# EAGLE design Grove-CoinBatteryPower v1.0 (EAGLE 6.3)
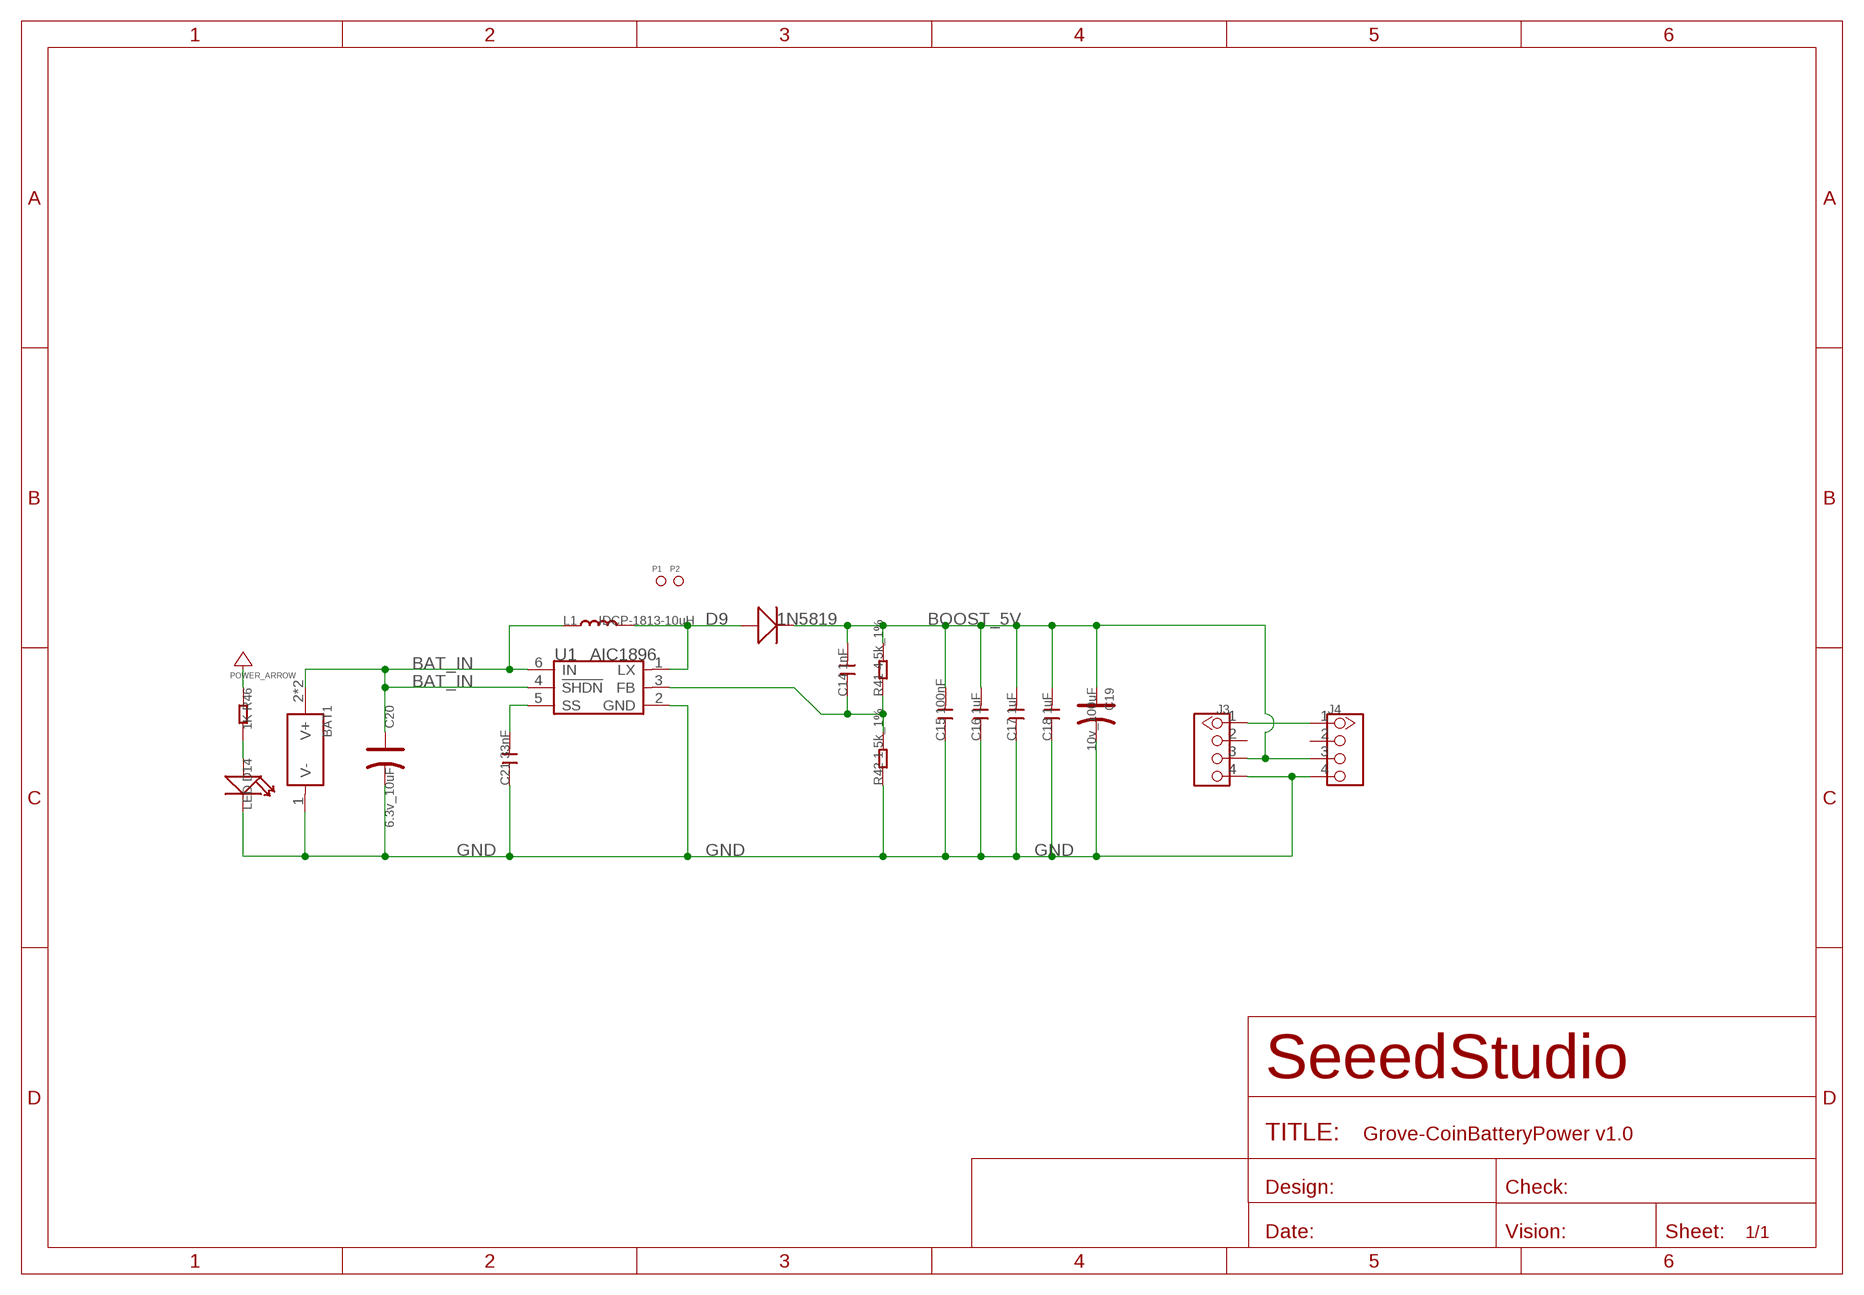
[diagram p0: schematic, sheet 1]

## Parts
BAT1  HOLDER-BAT-CIRCLE  [2032-D20-CIRCLE]
C14  1nF  C-0603  [C0603]
C15  100nF  C-0603  [C0603]
C16  1uF  C-0805  [C0805]
C17  1uF  C-0805  [C0805]
C18  1uF  C-0805  [C0805]
C19  10v_100uF  006-CAP_AVX_C  [AVX_C]
C20  6.3v_10uF  CAP-AVX-A  [AVX-A]
C21  33nF  C-0603  [C0603]
D9  1N5819  D'SMA'  [D2010]
D14  LED  LED'0603'  [LED-0603]
J3  TWIG-4P-2.0'90D'  [4P-2.0-90D]
J4  TWIG-4P-2.0'90D'  [4P-2.0-90D]
L1  IDCP-1813-10uH  013-L1813  [1813@1]
P1  PAD-MARK  [ROUND-MARK-1.0]
P2  PAD-MARK  [ROUND-MARK-1.0]
R41  4.5k_1%  R-0603  [R0603]
R42  1.5k_1%  R-0603  [R0603]
R46  1K  R-0603  [R0603]
U1  AIC1896  [SOT23-6]

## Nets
BAT_IN: BAT1.2(V+) BAT1.3(V+) C20.+ L1.1 U1.4(!SHDN) U1.6(IN)
BOOST_5V: C14.2 C15.2 C16.2 C17.2 C18.2 C19.+ D9.- J3.3 J4.3 R41.2 R46.1 ; supply symbol labelled POWER_ARROW
GND: BAT1.1(V-) C15.1 C16.1 C17.1 C18.1 C19.- C20.- C21.1 D14.- J3.4 J4.4 R42.1 U1.2(GND)
N$3: J3.1 J4.1
N$35: C21.2 U1.5(SS)
N$36: D9.+ L1.2 U1.1(LX)
N$37: C14.1 R41.1 R42.2 U1.3(FB)
N$74: D14.+ R46.2
Unconnected: J3.2 J4.2

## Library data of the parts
BAT1 = Connector:HOLDER-BAT: button cell holder
C14-C18 C21 = Discrete:C*: Ceramic Capacitors
C19 = Discrete:006-CAP*: Electrolytic Capacitors,Tantalum Capacitors and Super Capacitors
C20 = Discrete:CAP*: Electrolytic Capacitors,Tantalum Capacitors and Super Capacitors
D9 = Discrete:D*
D14 = Discrete:LED*
J3 J4 = Connector:TWIG-4P-2.0
L1 = Discrete:013-L*
P1 P2 = Discrete:PAD-MARK; PARTNO: DNP
R41 R42 R46 = Discrete:R*
U1 = ICs_v54:AIC1896

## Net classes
0 default: width 0.152 mm, drill 0.305 mm, clearance 0.152 mm

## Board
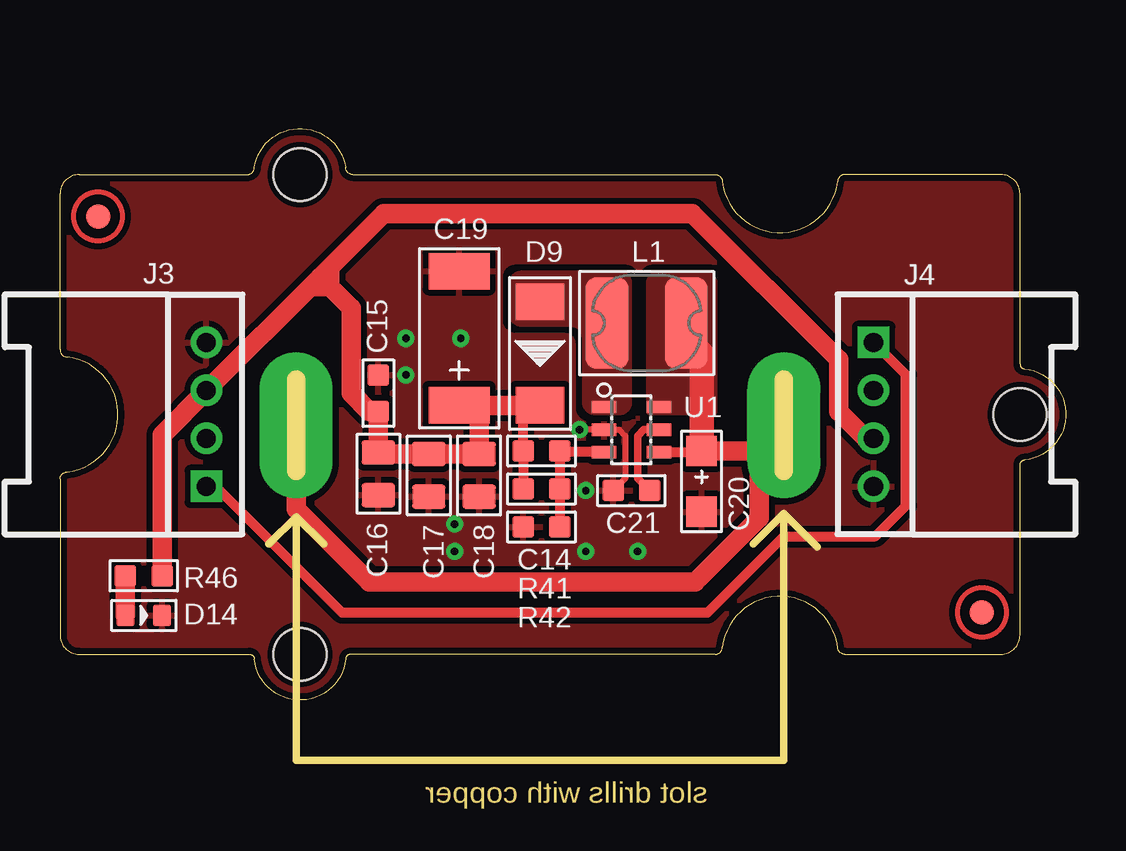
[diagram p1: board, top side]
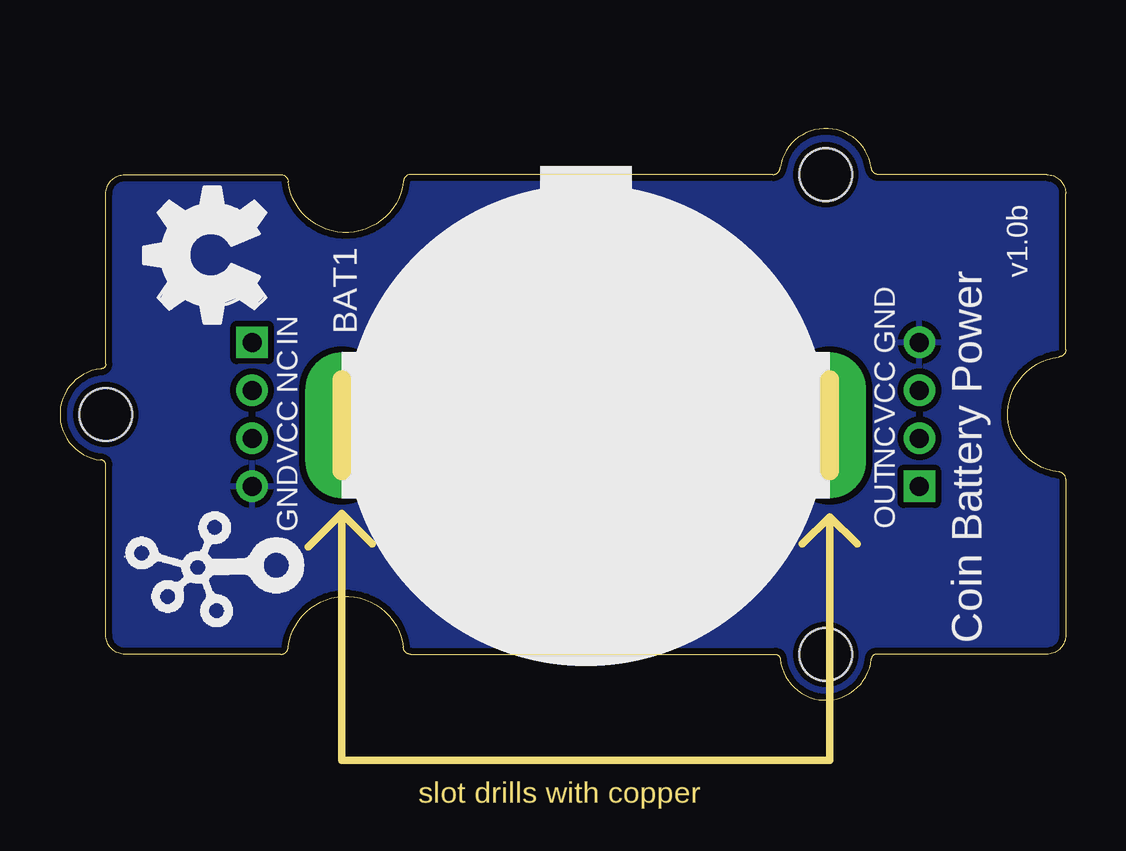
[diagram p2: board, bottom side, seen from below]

Size 41.91 x 23.83 mm. Coordinates in mm from the lower left corner, seen from the top.
Copper layers (1*16): Top 0.035mm / dielectric 1.5mm / Bottom 0.035mm
Design rules "default *": minimum track width 10mil, minimum drill 12mil, track to track 8mil, track to pad 8mil, pad to pad 8mil, via to via 8mil, smd to smd 0mil, copper to edge 10mil, drill to drill 8mil, minimum pad ring 10mil, minimum via ring 8mil, stop-mask expansion 4mil, vias tented up to drill 25mil, thermal gap 10mil

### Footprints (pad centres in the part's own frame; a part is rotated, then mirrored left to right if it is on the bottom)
2032-D20-CIRCLE = smd 15.24 x 15.24: 1 0,0 | drill 0.762 pad 3.048 long: 2 -10.16,0; 3 10.16,0
C0603 = smd 0.889 x 0.889: 1 -0.762,0; 2 0.762,0
C0805 = smd 1.016 x 1.397: 1 -0.889,0; 2 0.889,0
AVX_C = smd 1.524 x 2.54: + -2.794,0; - 2.794,0
AVX-A = smd 1.27 x 1.27: + -1.27,0; - 1.27,0
D2010 = smd 1.524 x 2.032: + -2.159,0; - 2.159,0
LED-0603 = smd 0.762 x 0.889: + -0.762,0; - 0.762,0
4P-2.0-90D = drill 0.8 pad 1.27 square: 1 -3,0 | drill 0.8 pad 1.27: 2 -1,0; 3 1,0; 4 3,0
1813@1 = smd 1.778 x 3.81: 1 -1.651,0; 2 1.651,0
ROUND-MARK-1.0 = smd 1.016 x 1.016: P$1 0,0
R0603 = smd 0.889 x 0.889: 1 -0.762,0; 2 0.762,0
SOT23-6 = smd 0.508 x 1.016: 1 -0.94,-1.143; 2 0,-1.143; 3 0.94,-1.143; 4 0.94,1.143; 5 0,1.143; 6 -0.94,1.143
2U-DIM-W/DRILL = hole 2.2: -10,-10; -10,10; 20,0

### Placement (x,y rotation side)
BAT1  20,11.45 0 bottom
C14  20.06,10.38 180 top
C15  13.27,12.8 270 top
C16  13.27,9.43 90 top
C17  15.36,9.37 90 top
C18  17.46,9.37 90 top
C19  16.63,15.08 90 top
C20  26.73,9.11 270 top
C21  23.81,8.73 0 top
D9  20,14.45 270 top
D14  3.49,3.53 0 top
J3  6.1,11.91 90 top
J4  33.9,11.91 270 top
L1  24.45,15.72 180 top
P1  1.59,20.16 0 top
P2  38.41,3.65 0 top
R41  20.06,8.8 180 top
R42  20.06,7.21 0 top
R46  3.49,5.18 180 top
U1  23.81,11.27 270 top
U$3  [OSHW_FILLX200_NOTEXT]  33.34,15.72 90 bottom
U$4  [TWIGLOGO]  32.7,5.56 90 bottom
U$6  [2U-DIM-W/DRILL]  20,11.91 0 top

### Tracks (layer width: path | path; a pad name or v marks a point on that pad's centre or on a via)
BAT_IN
  Top 0.406: U1.4 26.68,10.33 C20.+
  Top 0.813: C20.+ 29.09,10.38 | 29.09,10.38 BAT1.2 | BAT1.3 9.84,7.97 12.89,4.92 26.48,4.92 29.14,7.59 29.14,10.33 29.09,10.38
  Top 1.016: C20.+ 26.73,14.45 26.1,15.08 26.1,15.59 26.22,15.72
  pour Top (isolate 0.254, no thermals): 24.57,12.04 27.24,12.04 27.24,17.37 arc90 26.86,17.75 24.95,17.75 arc90 24.57,17.37
BOOST_5V
  Top 0.406: D9.- 19.3,11.59 C14.2 R41.2
  Top 0.813: D9.- 17.46,12.29 | 17.46,12.29 C19.+ | 17.46,12.29 C18.2 C17.2 13.33,10.26 C16.2 C15.2 12.89,12.04 12.13,12.8 12.13,16.35 11.24,17.24 | R46.1 4.25,11.06 J3.3 10.84,17.64 | J4.3 33.57,10.91 32.45,12.04 32.45,14.19 26.35,20.29 13.48,20.29 10.84,17.64 | 11.24,17.24 10.84,17.64 | 11.24,17.24 11.24,18 | 11.24,17.24 10.47,17.24
GND  (via drill 0.3 pad 0.64)
  Top 0.254: C21.1 23.56,9.24 23.56,11.02 23.3,11.27 U1.2 v21.65,11.27
  Bottom 0.254: v21.65,11.27 U1.2
  Bottom 0.305: v21.65,11.27 21.65,11.91 18.73,14.83 | 21.52,11.27 20.18,11.27 BAT1.1 | v16.7,15.08 17.71,15.08 18.22,14.58
  Bottom 0.406: v21.65,11.27 21.52,11.27 18.22,14.58
  other vias: 14.41,15.08 21.91,6.19 24.06,6.19 16.44,6.19 14.41,13.56 21.91,8.73 16.44,7.34
  pour Top (isolate 0.254, rank 6): -0.32,23.97 42.23,23.97 42.23,-0.16 -0.32,-0.16
  pour Bottom (isolate 0.254, rank 6): -0.32,23.97 42.23,23.97 42.23,-0.16 -0.32,-0.16
N$3
  Top 0.406: J3.1 6.49,8.91 11.74,3.65 26.98,3.65 30.16,6.83 33.97,6.83 35.24,8.1 35.24,13.57 J4.1
N$35
  Top 0.305: U1.5 24.32,11.27 24.06,11.02 24.06,9.24 C21.2
N$36
  pour Top (isolate 0.254, no thermals): 21.91,15.08 21.91,12.42 arc90 22.29,12.04 23.3,12.04 arc90 23.68,12.42 23.68,17.37 arc90 23.3,17.75 19.24,17.75 arc90 18.86,17.37 18.86,16.1 arc90 19.24,15.72 21.27,15.72 arc-90
N$37
  Top 0.406: U1.3 20.88,10.33 C14.1 R41.1 R42.2
N$74
  Top 0.813: D14.+ R46.2

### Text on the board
bPlace: v1.0b | GND | IN | NC | VCC | NC | VCC | OUT | GND | Coin Battery Power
